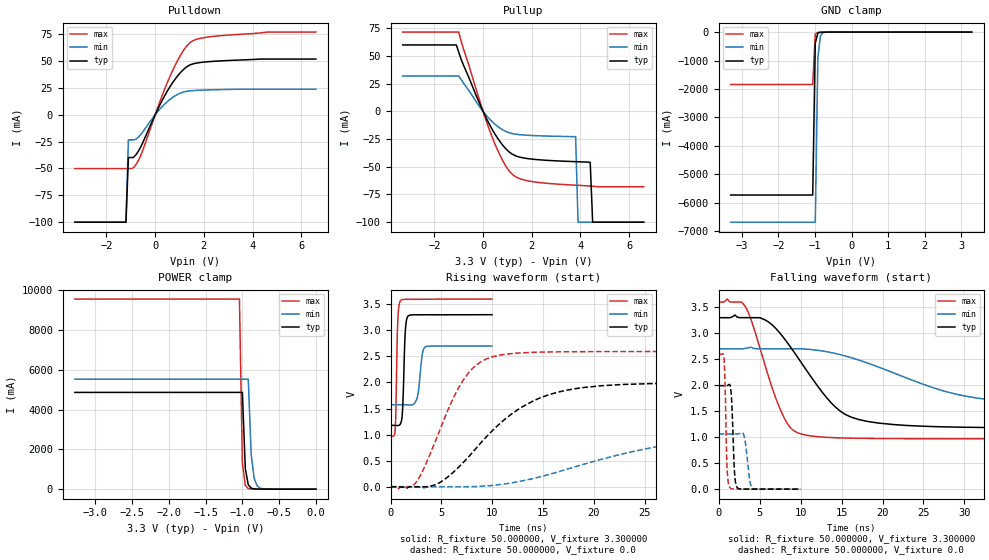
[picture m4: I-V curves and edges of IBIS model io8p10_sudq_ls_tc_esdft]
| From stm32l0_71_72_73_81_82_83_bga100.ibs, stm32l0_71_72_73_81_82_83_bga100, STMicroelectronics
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|   Model io8p10_sudq_ls_tc_esdft
[Model]  io8p10_sudq_ls_tc_esdft
Model_type I/O
Polarity   Non-Inverting
Enable   Active-Low
Vinl =   0.990000V
Vinh =   2.310000V
Vmeas =  1.650000V
Cref =   50.000000pF
Rref =   100.000000M
Vref =   0.0V
C_comp   2.248300pF   2.207300pF   2.311900pF
[Temperature Range]   25.000000   0.125000k   -40.000000
[Pullup Reference]   3.300000V   2.700000V   3.600000V
[Pulldown Reference]   0.0V   0.0V   0.0V
[POWER Clamp Reference]   3.300000V   2.700000V   3.600000V
[GND Clamp Reference]   0.0V   0.0V   0.0V
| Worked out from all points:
|   slope of the pulldown table from 0 to 0.495 V, typ, clamps not added: 22.6 ohm
|   slope of the pullup table from 0 to 0.495 V, typ, clamps not added: 23.9 ohm
|   GND clamp passes 1 mA (typ) near -0.64 V on its own axis
|   POWER clamp passes 1 mA (typ) near -0.63 V on its own axis
|   rising waveform, R_fixture 50.000000, V_fixture 3.300000: 20-80 % time 208ps typ, 363ps min, 164ps max; typ from 1.18 V to 3.3 V
|   rising waveform, R_fixture 50.000000, V_fixture 0.0: 20-80 % time 6.73ns typ, 13.7ns min, 3.61ns max; typ from 0 V to 1.99 V
|   falling waveform, R_fixture 50.000000, V_fixture 3.300000: 20-80 % time 5.99ns typ, 12.6ns min, 3.28ns max; typ from 3.3 V to 1.18 V
|   falling waveform, R_fixture 50.000000, V_fixture 0.0: 20-80 % time 290ps typ, 460ps min, 228ps max; typ from 1.99 V to 0 V
[Pulldown]
|Voltage   I(typ)   I(min)   I(max)
-3.3V     -100mA     -100mA     -50.11mA
-1.2V     -100mA     -100mA     -50.11mA
-1.1V     -39.8mA    -23.38mA   -50.11mA
-900mV    -39.8mA    -23.38mA   -49.43mA
-600mV    -30.26mA   -18.59mA   -38.38mA
500mV     22.11mA    12.28mA    30.06mA
900mV     35.58mA    18.71mA    49.62mA
1.3V      44.73mA    21.88mA    64.23mA
1.7V      48.13mA    22.72mA    70.3mA
2.4V      49.79mA    23.3mA     73.03mA
4.6V      51.9mA     23.82mA    77mA
6.6V      51.9mA     23.82mA    77mA
[Pullup]
|Voltage   I(typ)   I(min)   I(max)
-3.3V     60mA       32mA       71.6mA
-1.1V     60mA       32mA       71.6mA
-1V       53.5mA     32mA       71.6mA
-100mV    4.893mA    2.926mA    6.861mA
400mV     -17.21mA   -9.813mA   -24.69mA
900mV     -32.92mA   -17.72mA   -48.15mA
1.3V      -39.75mA   -20.41mA   -58.47mA
3.8V      -45.36mA   -22.8mA    -66.6mA
3.9V      -45.44mA   -100mA     -66.72mA
4.4V      -46mA      -100mA     -67.4mA
4.5V      -100mA     -100mA     -67.56mA
6.6V      -100mA     -100mA     -68mA
[GND_clamp]
|Voltage   I(typ)   I(min)   I(max)
-3.3V     -5.732A    -6.688A    -1.842A
-1.06V    -5.732A    -6.688A    -1.842A
-990mV    -389.4mA   -6.688A    -68.34mA
-920mV    -32.57mA   -918.2mA   -10.72mA
-850mV    -6.763mA   -131mA     -6.509mA
-780mV    -3.471mA   -21mA      -4.208mA
3.28V     0A         0A         0A
[POWER_clamp]
|Voltage   I(typ)   I(min)   I(max)
-3.28V    4.87A      5.538A     9.569A
-1.04V    4.87A      5.538A     9.569A
-1V       4.87A      5.538A     1.315A
-960mV    1.032A     5.538A     186.5mA
-920mV    222.2mA    5.538A     31.64mA
-880mV    50.73mA    1.734A     9.582mA
-840mV    13.93mA    544.8mA    5.668mA
-800mV    5.556mA    172.7mA    4.276mA
-760mV    3.231mA    55.84mA    3.297mA
-680mV    1.597mA    6.983mA    1.741mA
0V        0A         0A         0A
[Ramp]
| variable   typ   min   max
dV/dt_r  1.19496/6.71793n   0.62718/13.67013n   1.55568/3.60145n
dV/dt_f  1.27356/5.98091n   0.65286/12.48000n   1.57788/3.27566n
R_load = 50.000000
[Rising Waveform]
R_fixture= 50.000000
V_fixture= 3.300000
V_fixture_min= 2.700000
V_fixture_max= 3.600000
|time   V(typ)   V(min)   V(max)
0s        1.177V     1.573V     970.2mV
440.4ps   1.176V     1.573V     1.085V
680.7ps   1.173V     1.573V     3.097V
961ps     1.207V     1.573V     3.568V
1.181ns   1.517V     1.573V     3.591V
1.441ns   2.991V     1.572V     3.595V
1.722ns   3.275V     1.569V     3.595V
2.603ns   3.298V     1.706V     3.595V
3.383ns   3.299V     2.679V     3.597V
9.97ns    3.3V       2.7V       3.6V
[Rising Waveform]
R_fixture= 50.000000
V_fixture= 0.0
V_fixture_min= 0.0
V_fixture_max= 0.0
|time   V(typ)   V(min)   V(max)
0s        8.068uV    -5.322uV   362.8uV
2.503ns   -1.405mV   -3.573mV   85.64mV
4.805ns   76.52mV    -561.7uV   1.071V
6.907ns   416.9mV    -394.9uV   1.97V
8.308ns   714.7mV    2.421mV    2.315V
10.01ns   1.076V     23.08mV    2.492V
14.01ns   1.643V     156.3mV    2.578V
19.02ns   1.904V     430.5mV    2.591V
30.83ns   1.989V     898.2mV    2.593V
49.85ns   1.992V     1.062V     2.593V
[Falling Waveform]
R_fixture= 50.000000
V_fixture= 3.300000
V_fixture_min= 2.700000
V_fixture_max= 3.600000
|time   V(typ)   V(min)   V(max)
0s        3.3V       2.7V       3.6V
3.303ns   3.3V       2.71V      3.502V
5.706ns   3.254V     2.7V       2.365V
7.508ns   2.998V     2.7V       1.542V
8.709ns   2.748V     2.7V       1.193V
9.91ns    2.476V     2.7V       1.07V
14.11ns   1.6V       2.616V     990.4mV
18.22ns   1.302V     2.424V     976.4mV
31.33ns   1.189V     1.757V     970.5mV
49.85ns   1.177V     1.573V     970.2mV
[Falling Waveform]
R_fixture= 50.000000
V_fixture= 0.0
V_fixture_min= 0.0
V_fixture_max= 0.0
|time   V(typ)   V(min)   V(max)
0s        1.992V     1.062V     2.593V
660.7ps   1.992V     1.062V     2.515V
1.021ns   1.993V     1.062V     452.7mV
1.341ns   2.014V     1.062V     39.58mV
1.582ns   1.724V     1.062V     9.014mV
1.962ns   278.8mV    1.062V     3.591mV
2.282ns   28.21mV    1.062V     3.156mV
3.103ns   1.568mV    1.027V     2.895mV
4.124ns   1.062mV    22.83mV    2.676mV
9.97ns    8.068uV    -5.322uV   362.8uV
